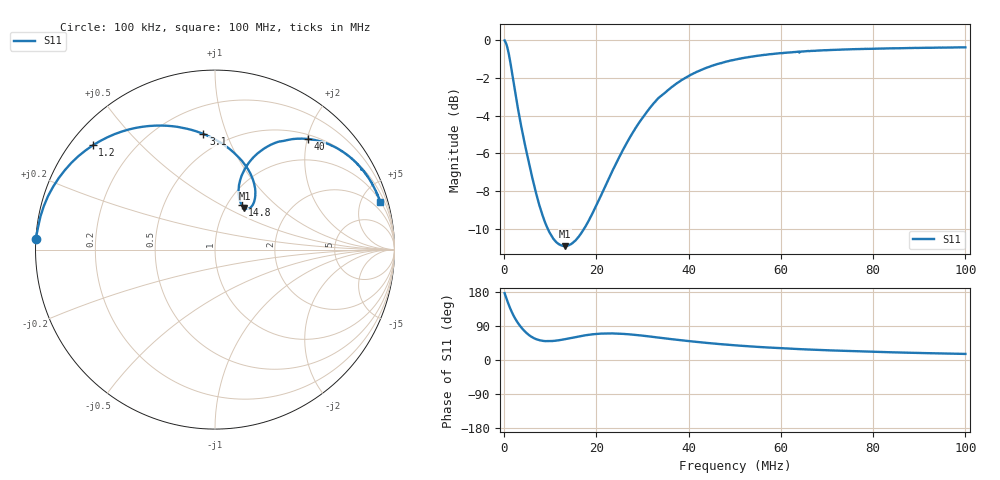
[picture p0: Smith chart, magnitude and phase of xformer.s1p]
# Hz S RI R 50.0
! written by SimSmith version 18.3h
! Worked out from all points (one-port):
!   1000 points, 100 kHz to 100 MHz, reference 50 ohm
!   lowest |S11| = -10.9 dB at 13.1 MHz (marker M1), VSWR 1.79, Z = 61 + j30.8 ohm
!   |S11| at or under -10 dB: 9.427 MHz to 17.35 MHz (7.924 MHz wide, 59.2 % of centre)
!   S11 on the Smith chart (normalised r, x): 100 kHz: -0.00, +0.03; 1.2 MHz: 0.06, +0.37; 3.1 MHz: 0.37, +0.83; 14.8 MHz: 1.17, +0.63; 40 MHz: 0.58, +2.01; 100 MHz: 1.06, +6.94
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100000  -0.9982 0.0615
600000  -0.9017 0.3505
900000  -0.7997 0.4839
1200000  -0.6809 0.581
1600000  -0.5182 0.6581
2000000  -0.3679 0.6886
2500000  -0.2096 0.684
3100000  -0.0642 0.6446
3700000  0.0404 0.5902
4400000  0.1247 0.5217
5200000  0.1843 0.4471
6000000  0.2143 0.3811
7300000  0.2249 0.3031
8800000  0.2119 0.253
1.07e7  0.189 0.2287
1.26e7  0.1688 0.2293
1.31e7  0.1637 0.232
1.48e7  0.1496 0.2474
2.04e7  0.1329 0.3492
2.51e7  0.1734 0.462
3.17e7  0.3138 0.5856
3.76e7  0.462 0.618
4e7  0.5176 0.616
5.01e7  0.6941 0.5566
6.26e7  0.8098 0.4587
7.51e7  0.8685 0.3783
8.76e7  0.9008 0.3147
1e8  0.9214 0.2649
